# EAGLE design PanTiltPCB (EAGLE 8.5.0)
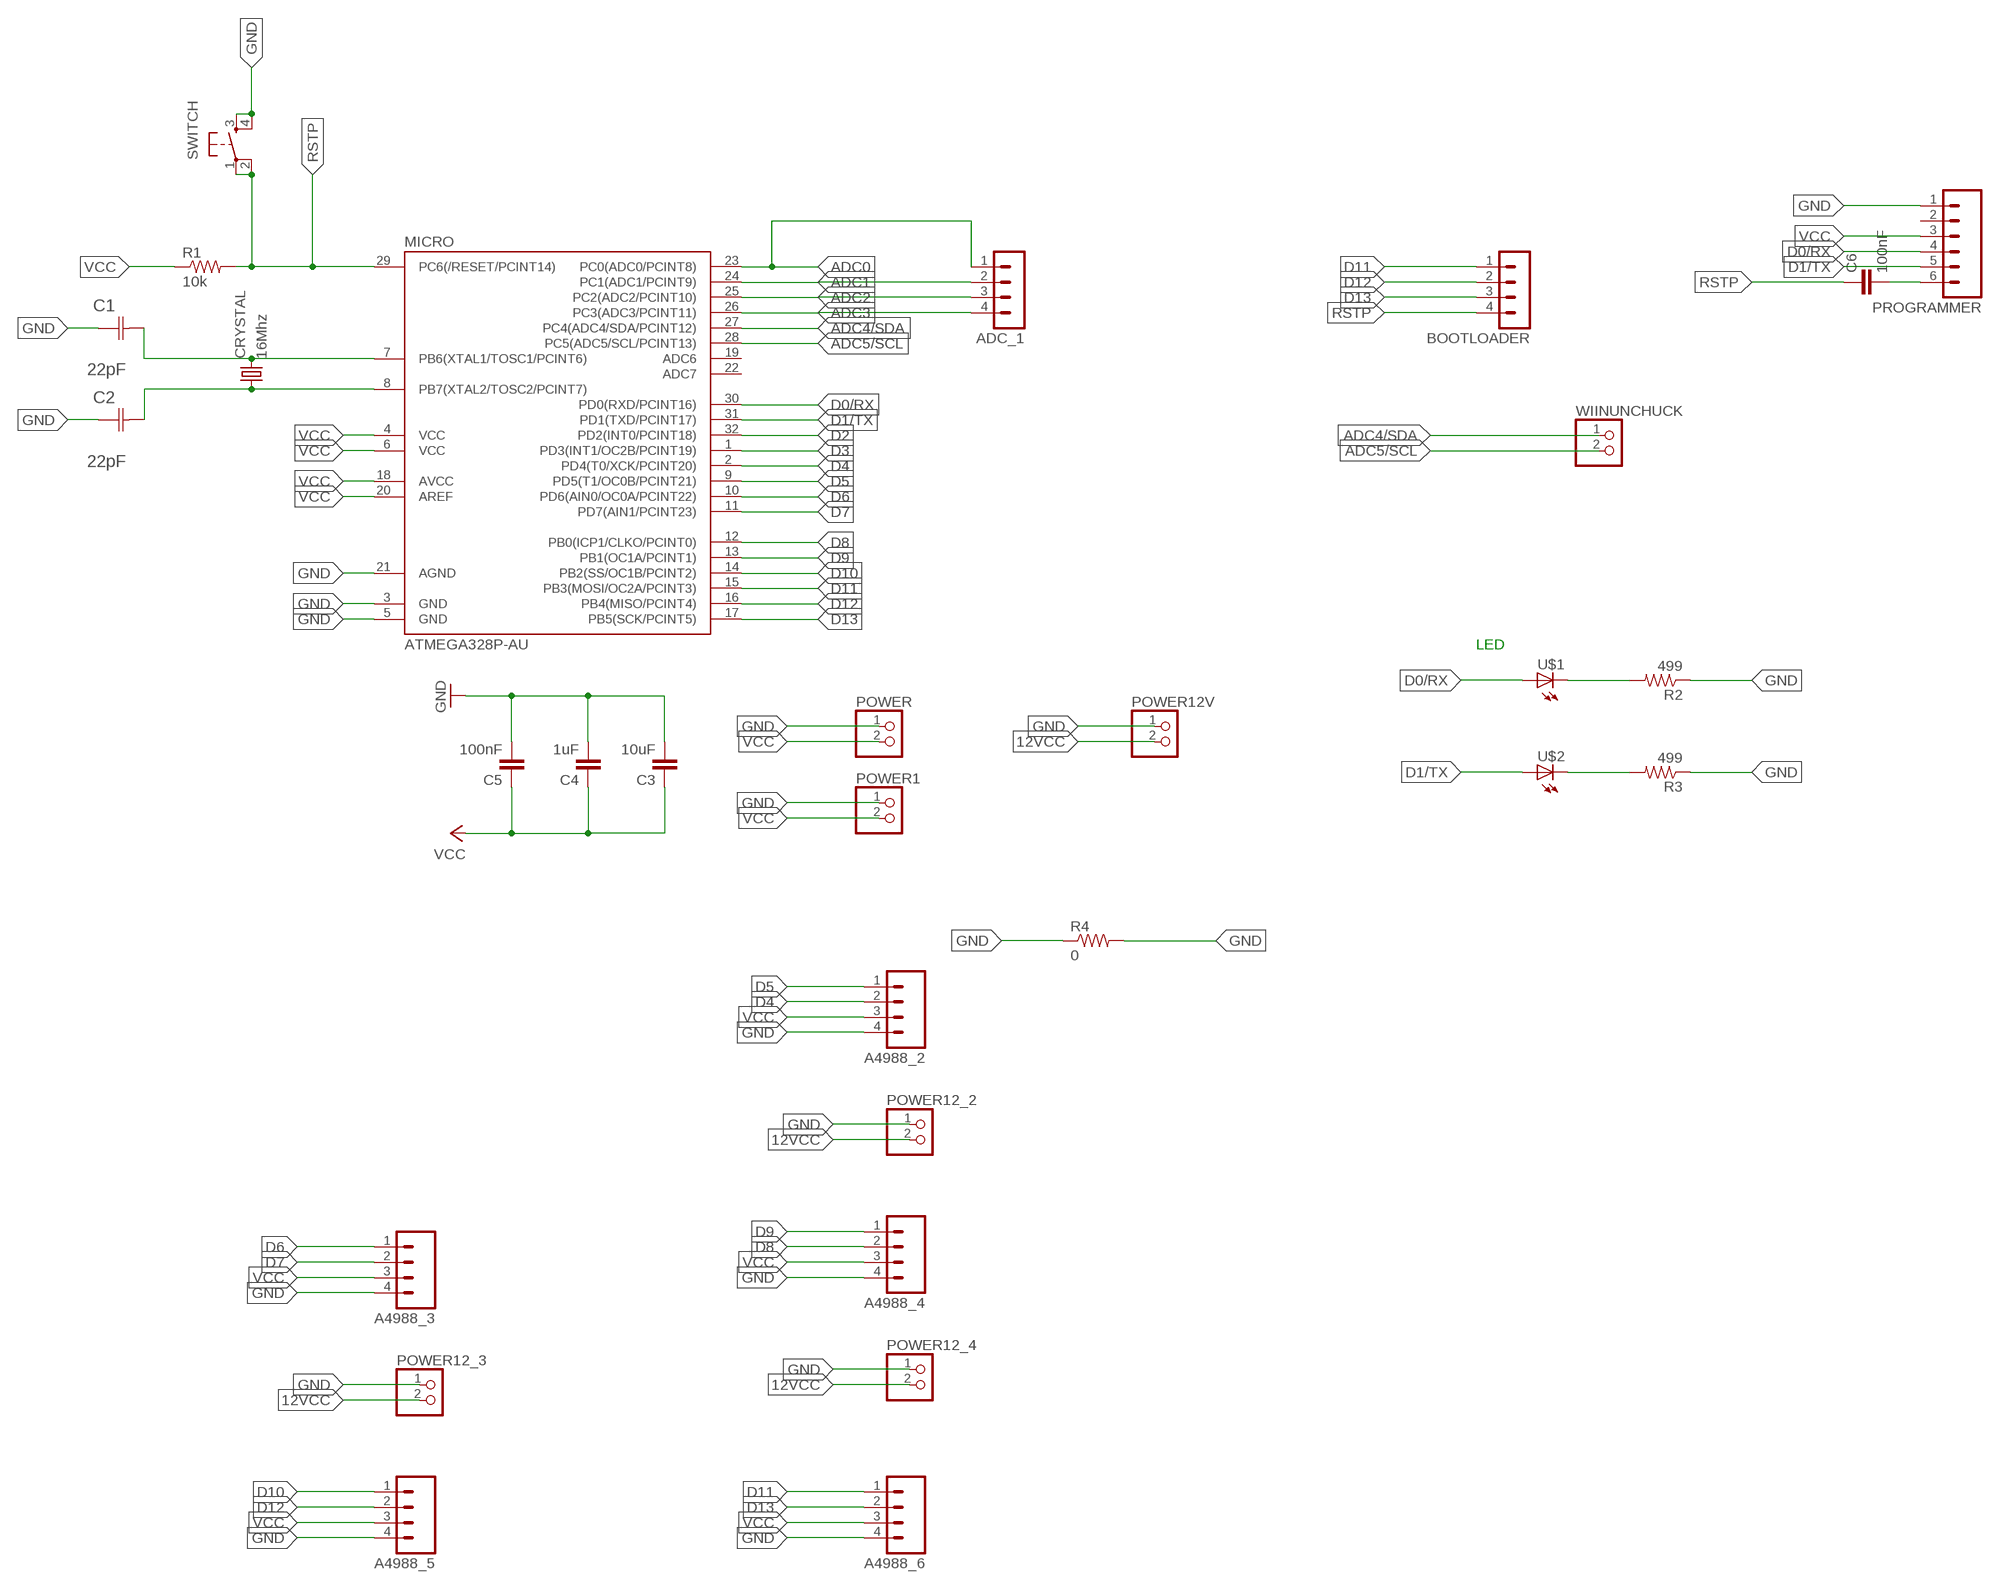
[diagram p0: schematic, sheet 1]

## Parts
A4988_2  M04  [04P]
A4988_3  M04  [04P]
A4988_4  M04  [04P]
A4988_5  M04  [04P]
A4988_6  M04  [04P]
ADC_1  MA04-1  [MA04-1]
BOOTLOADER  MA04-1  [MA04-1]
C1  22pF  0612ZC225MAT2A  [CAPC3216X178N]
C2  22pF  0612ZC225MAT2A  [CAPC3216X178N]
C3  10uF  CAP1206  [1206]
C4  1uF  CAP1206  [1206]
C5  100nF  CAP1206  [1206]
C6  100nF  CAP1206  [1206]
CRYSTAL  16Mhz  CSM-7X-DU  [CSM-7X-DU]
MICRO  ATMEGA328P-AU  ATMEGA48/88/168-AU  [TQFP32-08]
POWER  PINHD-1X2  [1X02]
POWER1  PINHD-1X2  [1X02]
POWER12_2  PINHD-1X2  [1X02]
POWER12_3  PINHD-1X2  [1X02]
POWER12_4  PINHD-1X2  [1X02]
POWER12V  PINHD-1X2  [1X02]
PROGRAMMER  M06  [06P]
R1  10k  RESISTOR1206  [1206]
R2  499  RESISTOR1206  [1206]
R3  499  RESISTOR1206  [1206]
R4  0  RESISTOR1206  [1206]
SWITCH  6MM_SWITCH6MM_SWITCH  [6MM_SWITCH]
U$1  LED1206  [1206]
U$2  LED1206  [1206]
WIINUNCHUCK  PINHD-1X2  [1X02]

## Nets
12VCC: POWER12_2.2 POWER12_3.2 POWER12_4.2 POWER12V.2
ADC0: ADC_1.1 MICRO.23(PC0(ADC0/PCINT8))
ADC1: ADC_1.2 MICRO.24(PC1(ADC1/PCINT9))
ADC2: ADC_1.3 MICRO.25(PC2(ADC2/PCINT10))
ADC3: ADC_1.4 MICRO.26(PC3(ADC3/PCINT11))
ADC4/SDA: MICRO.27(PC4(ADC4/SDA/PCINT12)) WIINUNCHUCK.1
ADC5/SCL: MICRO.28(PC5(ADC5/SCL/PCINT13)) WIINUNCHUCK.2
D0/RX: MICRO.30(PD0(RXD/PCINT16)) PROGRAMMER.4 U$1.1(A)
D1/TX: MICRO.31(PD1(TXD/PCINT17)) PROGRAMMER.5 U$2.1(A)
D2: MICRO.32(PD2(INT0/PCINT18))
D3: MICRO.1(PD3(INT1/OC2B/PCINT19))
D4: A4988_2.2 MICRO.2(PD4(T0/XCK/PCINT20))
D5: A4988_2.1 MICRO.9(PD5(T1/OC0B/PCINT21))
D6: A4988_3.1 MICRO.10(PD6(AIN0/OC0A/PCINT22))
D7: A4988_3.2 MICRO.11(PD7(AIN1/PCINT23))
D8: A4988_4.2 MICRO.12(PB0(ICP1/CLKO/PCINT0))
D9: A4988_4.1 MICRO.13(PB1(OC1A/PCINT1))
D10: A4988_5.1 MICRO.14(PB2(SS/OC1B/PCINT2))
D11: A4988_6.1 BOOTLOADER.1 MICRO.15(PB3(MOSI/OC2A/PCINT3))
D12: A4988_5.2 BOOTLOADER.2 MICRO.16(PB4(MISO/PCINT4))
D13: A4988_6.2 BOOTLOADER.3 MICRO.17(PB5(SCK/PCINT5))
GND: A4988_2.4 A4988_3.4 A4988_4.4 A4988_5.4 A4988_6.4 C1.1(C1) C2.1(C1) C3.2 C4.2 C5.2 MICRO.3(GND) MICRO.5(GND) MICRO.21(AGND) POWER1.1 POWER12_2.1 POWER12_3.1 POWER12_4.1 POWER12V.1 POWER.1 PROGRAMMER.1 R2.1 R3.1 R4.1 R4.2 SWITCH.3(S) SWITCH.4(S1)
N$1: C6.2 PROGRAMMER.6
N$2: C1.2(C2) CRYSTAL.2 MICRO.7(PB6(XTAL1/TOSC1/PCINT6))
N$9: C2.2(C2) CRYSTAL.1 MICRO.8(PB7(XTAL2/TOSC2/PCINT7))
N$39: R2.2 U$1.2(C)
N$40: R3.2 U$2.2(C)
RSTP: BOOTLOADER.4 C6.1 MICRO.29(PC6(/RESET/PCINT14)) R1.2 SWITCH.1(P) SWITCH.2(P1)
VCC: A4988_2.3 A4988_3.3 A4988_4.3 A4988_5.3 A4988_6.3 C3.1 C4.1 C5.1 MICRO.4(VCC) MICRO.6(VCC) MICRO.18(AVCC) MICRO.20(AREF) POWER1.2 POWER.2 PROGRAMMER.3 R1.1
Unconnected: MICRO.19(ADC6) MICRO.22(ADC7) PROGRAMMER.2

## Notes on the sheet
- LED

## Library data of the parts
A4988_2-A4988_6 = con-amp-quick:M04: AMP QUICK CONNECTOR; OC_FARNELL: unknown; OC_NEWARK: unknown
ADC_1 BOOTLOADER = con-lstb:MA04-1: PIN HEADER; OC_FARNELL: unknown; OC_NEWARK: unknown
C1 C2 = AVX_By_element14_Batch_1:0612ZC225MAT2A: Capacitor 1206; MPN: 0612ZC225MAT2A; OC_FARNELL: -; OC_NEWARK: 12N3209; SUPPLIER: AVX; TOLERANCE: ±20%; VALUE: 2.2µF; VOLTAGERATING: 10V
C3-C6 = 01_SparkFun:CAP: Capacitor
CRYSTAL = 01_FAB_Hello:CSM-7X-DU: SMD CRYSTAL; OC_FARNELL: unknown; OC_NEWARK: unknown
MICRO = atmega8:ATMEGA48/88/168
POWER POWER1 POWER12_2-POWER12_4 POWER12V WIINUNCHUCK = pinhead:PINHD-1X2: PIN HEADER
PROGRAMMER = con-amp-quick:M06: AMP QUICK CONNECTOR; OC_FARNELL: unknown; OC_NEWARK: unknown
R1 R4 = 01_SparkFun:RESISTOR: Resistor
R2 R3 = FAB_Hello:RESISTOR
SWITCH = 01_FAB_Hello:6MM_SWITCH: OMRON SWITCH
U$1 U$2 = FAB_Hello:LED

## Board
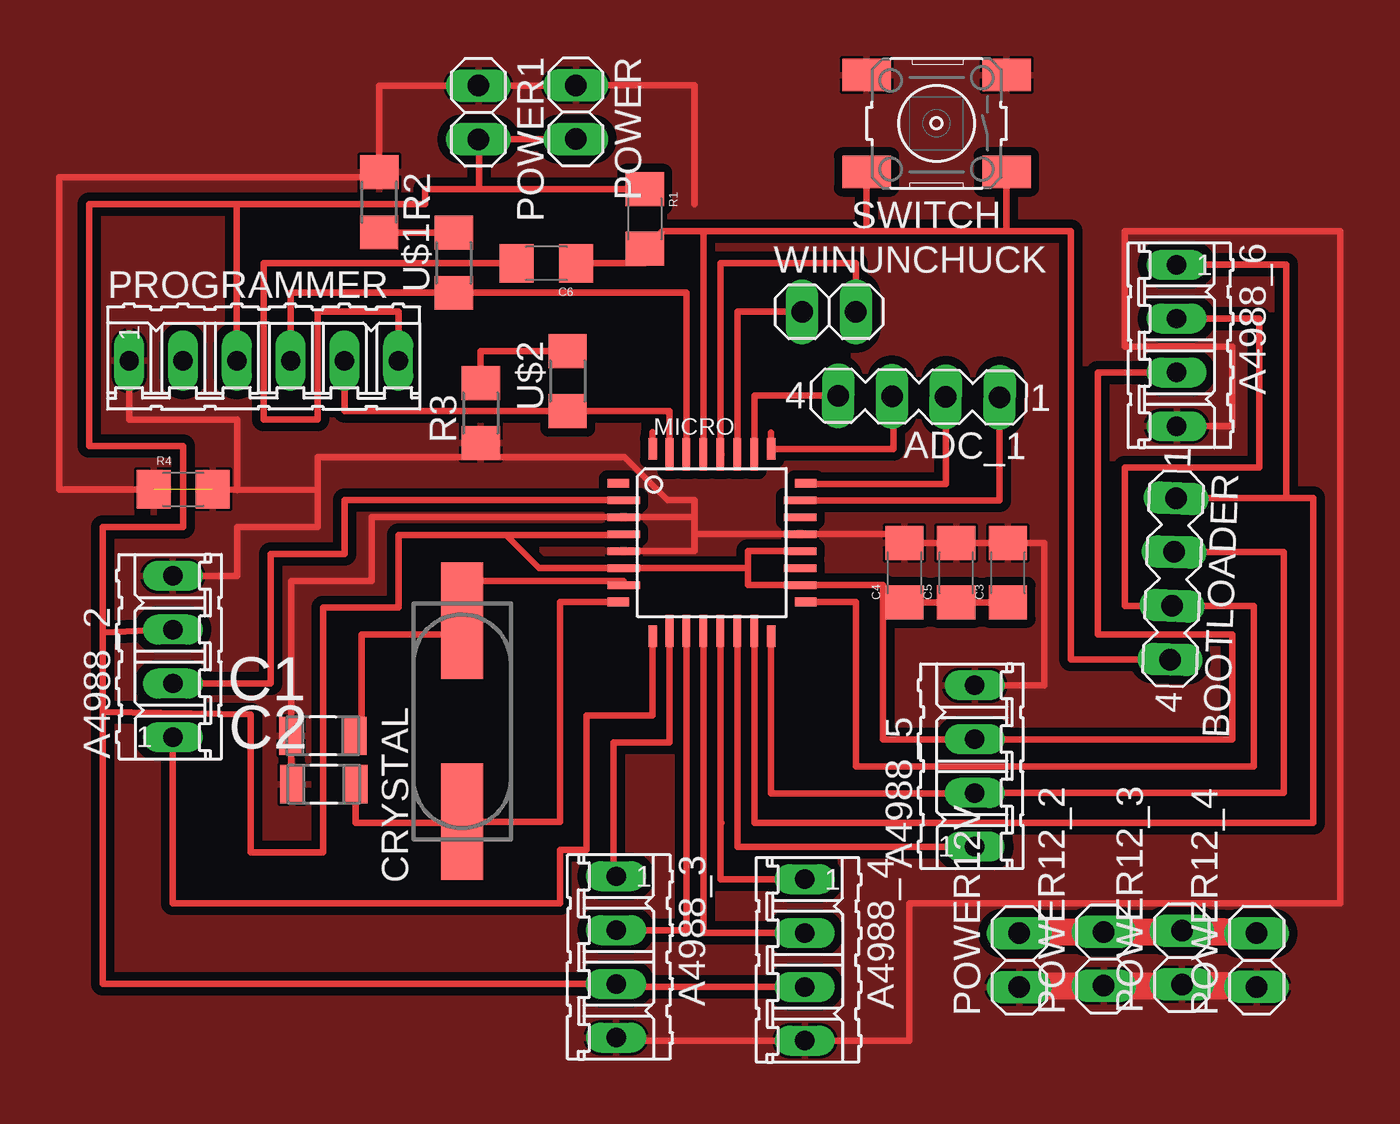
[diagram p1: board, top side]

No outline drawn. Coordinates in mm, seen from the top.
Copper layers (1*16): Top 0.035mm / dielectric 1.5mm / Bottom 0.035mm
Design rules "default *": minimum track width 10mil, minimum drill 24mil, track to track 8mil, track to pad 8mil, pad to pad 8mil, via to via 8mil, smd to smd 8mil, copper to edge 5mil, drill to drill 8mil, minimum pad ring 10mil, minimum via ring 8mil, stop-mask expansion 4mil, vias tented up to drill 0mil, thermal gap 5mil

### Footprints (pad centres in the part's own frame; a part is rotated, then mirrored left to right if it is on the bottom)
04P = drill 0.914 long: 1 -3.81,0; 2 -1.27,0; 3 1.27,0; 4 3.81,0
MA04-1 = drill 1.016 long: 1 -3.81,0; 2 -1.27,0; 3 1.27,0; 4 3.81,0
CAPC3216X178N = smd 1.118 x 1.803: 1 -1.499,0; 2 1.499,0
1206 = smd 1.6 x 1.8: 1 -1.4,0; 2 1.4,0
CSM-7X-DU = smd 5.5 x 2: 1 -4.75,0; 2 4.75,0
TQFP32-08 = smd 1.016 x 0.406: 1 -4.42,2.8; 8 -4.42,-2.8; 17 4.42,-2.8; 24 4.42,2.8 | smd 1.524 x 0.356: 2 -4.166,2; 3 -4.166,1.2; 4 -4.166,0.4; 5 -4.166,-0.4; 6 -4.166,-1.2; 7 -4.166,-2; 18 4.166,-2; 19 4.166,-1.2; 20 4.166,-0.4; 21 4.166,0.4; 22 4.166,1.2; 23 4.166,2 | smd 0.406 x 1.016: 9 -2.8,-4.42; 16 2.8,-4.42; 25 2.8,4.42; 32 -2.8,4.42 | smd 0.356 x 1.524: 10 -2,-4.166; 11 -1.2,-4.166; 12 -0.4,-4.166; 13 0.4,-4.166; 14 1.2,-4.166; 15 2,-4.166; 26 2,4.166; 27 1.2,4.166; 28 0.4,4.166; 29 -0.4,4.166; 30 -1.2,4.166; 31 -2,4.166
1X02 = drill 1.016 long: 1 -1.27,0; 2 1.27,0
06P = drill 0.914 long: 1 -6.35,0; 2 -3.81,0; 3 -1.27,0; 4 1.27,0; 5 3.81,0; 6 6.35,0
1206' = smd 1.6 x 1.803: 1 -1.422,0; 2 1.422,0
6MM_SWITCH = smd 2.286 x 1.524: 1 -3.302,2.286; 2 3.302,2.286; 3 -3.302,-2.286; 4 3.302,-2.286

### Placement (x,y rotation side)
A4988_2  31.26,31.98 90 top
A4988_3  52.19,17.8 270 top
A4988_4  61.09,17.66 270 top
A4988_5  69.11,26.81 90 top
A4988_6  78.64,46.67 270 top
ADC_1  66.48,44.25 179.4 top
BOOTLOADER  78.48,35.65 267.9 top
C1  38.34,28.24 0 top
C2  38.39,25.96 0 top
C3  70.68,35.94 90 top
C4  65.8,35.94 90 top
C5  68.24,35.94 90 top
C6  48.9,50.55 180 top
CRYSTAL  44.92,28.93 90 top
MICRO  56.71,37.36 0 top
POWER  50.28,57.68 270 top
POWER1  45.68,57.66 270 top
POWER12_2  75.21,17.71 90 top
POWER12_3  78.89,17.77 90 top
POWER12_4  82.42,17.65 90 top
POWER12V  71.22,17.65 90 top
PROGRAMMER  35.55,45.95 0 top
R1  53.54,52.64 270 top
R2  499  [1206']  41,53.43 269.8 top
R3  499  [1206']  45.8,43.48 90 top
R4  31.75,39.88 0 top
SWITCH  67.31,57.15 180 top
U$1  [1206']  44.52,50.57 90 top
U$2  [1206']  49.9,44.98 90 top
WIINUNCHUCK  62.23,48.26 0 top

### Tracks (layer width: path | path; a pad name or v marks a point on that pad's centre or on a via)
12VCC
  Top 1.27: POWER12V.2 71.22,18.98 POWER12_2.2 80.92,18.98 | 80.92,18.98 POWER12_3.2 | 80.92,18.98 82.42,18.98 POWER12_4.2
ADC0
  Top 0.305: MICRO.23 62.23,39.35 | 62.77,39.35 62.23,39.35 | 62.23,39.35 70.29,39.35 ADC_1.1
ADC1
  Top 0.305: MICRO.24 61.16,40.13 67.75,40.13 ADC_1.2
ADC2
  Top 0.305: MICRO.25 59.51,42.55 | 59.56,41.78 MICRO.25 | MICRO.25 65.28,41.78 65.28,44.27 ADC_1.3
ADC3
  Top 0.305: MICRO.26 58.71,44.29 ADC_1.4
ADC4/SDA
  Top 0.305: MICRO.27 57.91,48.26 WIINUNCHUCK.1
ADC5/SCL
  Top 0.305: 57.15,41.52 MICRO.28 57.11,50.55 63.5,50.55 WIINUNCHUCK.2
D0/RX
  Top 0.305: 36.9,45.95 PROGRAMMER.4 36.83,49.15 | 36.83,49.15 U$1.1 55.51,49.15 MICRO.30 | 36.83,49.15 36.82,49.15
D1/TX
  Top 0.305: 54.71,43.56 54.61,43.56 | 54.61,43.56 U$2.1 39.36,43.56 PROGRAMMER.5 | MICRO.31 54.71,43.46 54.61,43.56
D2
  Top 0.305: 53.91,42.57 MICRO.32
D4
  Top 0.305: MICRO.2 39.37,39.37 39.37,36.83 35.88,36.83 35.88,30.71 A4988_2.2
D5
  Top 0.305: A4988_2.1 31.26,20.32 49.53,20.32 49.53,22.86 50.8,22.86 50.8,29.21 53.91,29.21 MICRO.9
D6
  Top 0.305: MICRO.10 54.71,27.94 52.07,27.94 52.07,21.61 A4988_3.1
D7
  Top 0.305: MICRO.11 55.51,19.07 A4988_3.2
D8
  Top 0.305: MICRO.12 56.31,18.93 A4988_4.2
D9
  Top 0.305: MICRO.13 57.11,24.17 | 57.11,24.17 57.15,24.13 | 57.11,24.17 57.11,21.47 A4988_4.1
D10
  Top 0.305: A4988_5.1 69.11,22.99 57.91,22.99 MICRO.14
D11
  Top 0.305: 83.82,39.46 85.09,39.46 85.09,24.13 58.71,24.13 MICRO.15 | 83.82,39.46 BOOTLOADER.1 | A4988_6.1 83.82,50.48 83.82,39.46
D12
  Top 0.305: BOOTLOADER.2 83.69,36.92 83.69,25.54 A4988_5.2 69.11,25.53 59.51,25.53 MICRO.16
D13
  Top 0.305: BOOTLOADER.3 79.03,34.38 | MICRO.17 63.5,34.56 63.5,26.8 82.3,26.8 82.3,34.38 BOOTLOADER.3 | BOOTLOADER.3 76.2,34.38 76.2,40.89 82.55,40.89 82.55,47.94 A4988_6.2
GND  (1 unrouted)
  Top 0.305: MICRO.21 | MICRO.21 55.88,37.76 | 55.88,37.76 55.88,36.96 MICRO.5 | 55.88,38.56 MICRO.3 40.64,38.56 40.64,35.56 36.84,35.56 C1.1 36.84,25.95 C2.1 | 55.88,38.56 55.88,37.76 | MICRO.21 65.8,37.76 C4.2 C5.2 C3.2 72.39,37.34 72.39,30.62 A4988_5.4 | 55.88,38.56 55.88,39.37 54.61,39.37 52.58,41.4 45.72,41.4 | A4988_3.4 52.19,13.85 A4988_4.4 66.04,13.85 66.04,20.32 86.36,20.32 86.36,52.07 76.2,52.07 76.2,46.61 81.28,46.61 81.28,42.86 A4988_6.4 | 45.72,41.4 38.1,41.4 38.1,39.88 | R3.1 45.72,41.55 45.72,41.4 | R4.2 34.31,39.84 | 34.31,39.84 38.1,39.88 | R4.1 25.91,39.88 25.91,54.61 41.01,54.61 R2.1 41.01,58.94 POWER1.1 49.53,58.94 49.53,58.95 POWER.1 55.88,58.95 55.88,53.34 | A4988_2.4 34.29,35.79 34.29,38.1 38.1,38.1 38.1,39.88 | PROGRAMMER.1 29.21,43.18 34.29,43.18 34.29,39.84 34.31,39.84
  Top 1.27: POWER12V.1 71.22,16.44 POWER12_2.1 80.92,16.44 POWER12_3.1
  pour Top (isolate 0.406): 21.59,8.89 91.44,8.89 91.44,63.5 21.59,63.5
N$1
  Top 0.305: C6.2 45.72,50.55 35.56,50.55 35.56,43.18 38.1,43.18 38.1,48.26 41.91,48.26 PROGRAMMER.6
N$2
  Top 0.305: C1.2 40.17,28.24 40.17,33.02 44.92,33.02 CRYSTAL.2 44.92,35.56 | MICRO.7 52.54,35.56 44.92,35.56 | 44.45,35.56 44.92,35.56
N$9
  Top 0.305: MICRO.8 49.53,34.56 49.53,24.18 CRYSTAL.1 44.92,24.13 44.45,24.13 43.18,24.13 39.89,24.13 C2.2
N$39
  Top 0.305: U$1.2 44.51,52.01 R2.2
N$40
  Top 0.305: R3.2 45.8,46.41 U$2.2
RSTP
  Top 0.305: C6.1 53.54,50.55 R1.2 54.36,52.06 56.31,52.06 | MICRO.29 56.31,52.06 | 64.01,52.06 66.04,52.06 66.04,52.07 70.61,52.07 | 64.01,52.06 56.31,52.06 | 70.61,52.07 73.66,52.07 73.66,31.84 BOOTLOADER.4 | SWITCH.1 70.61,52.07 | SWITCH.2 64.01,52.06
VCC
  Top 0.254: MICRO.4 52.7,37.76
  Top 0.305: MICRO.18 | 60.87,35.33 MICRO.18 | 67.46,34.4 C5.1 | 46.99,37.72 41.91,37.72 41.91,34.29 38.35,34.29 38.35,22.73 34.92,22.73 34.92,29.24 27.96,29.37 | 46.99,37.72 52.66,37.72 52.7,37.76 | 27.96,33.12 27.96,38.1 31.75,38.1 31.75,41.91 27.3,41.91 27.3,53.34 34.28,53.34 | 27.96,33.12 27.96,29.37 | 27.96,29.37 27.96,16.53 A4988_3.3 52.19,16.39 A4988_4.3 | 46.99,37.72 48.55,36.16 MICRO.6 58.42,36.16 | MICRO.18 58.42,35.36 58.42,36.16 | MICRO.20 58.42,36.96 58.42,36.16 | A4988_2.3 27.96,33.12 | C3.1 C5.1 | 53.54,53.85 R1.1 45.72,54.04 | MICRO.18 64.77,35.36 64.77,34.29 | 64.77,34.29 65.8,34.29 C4.1 C5.1 | 64.77,34.29 64.77,28.08 A4988_5.3 81.28,28.08 81.28,33.02 74.93,33.02 74.93,45.4 A4988_6.3 | PROGRAMMER.3 34.28,53.34 | 45.72,54.04 43.18,54.04 43.18,53.34 34.28,53.34 | 45.72,54.04 45.72,56.4 POWER1.2 49.01,56.4 POWER.2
